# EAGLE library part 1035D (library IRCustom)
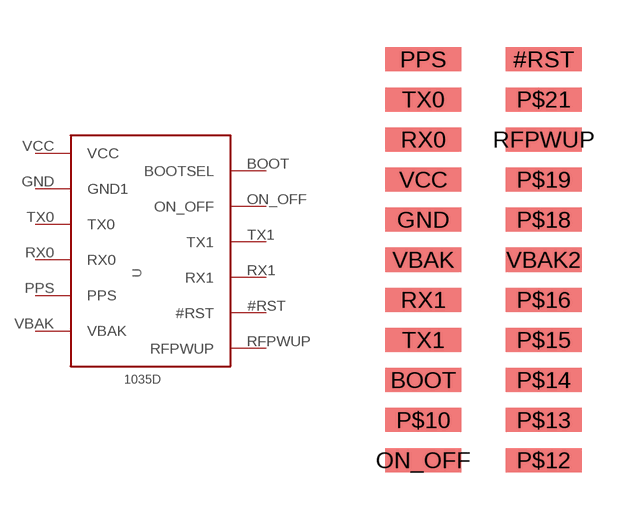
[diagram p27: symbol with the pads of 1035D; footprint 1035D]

Designator prefix -

## 1035D  [1035D]
#RST  #RST  in
BOOT  BOOTSEL  in
GND  GND1  sup
ON_OFF  ON_OFF  in
PPS  PPS  out
RFPWUP  RFPWUP  out
RX0  RX0  in
RX1  RX1  in
TX0  TX0  out
TX1  TX1  out
VBAK  VBAK  sup
VCC  VCC  sup

## Footprint 1035D (pad centres in mm)
smd 2.4 x 0.76: #RST 16.96,6.39; BOOT 13.15,-3.77; GND 13.15,1.31; ON_OFF 13.15,-6.31; P$10 13.15,-5.04; P$12 16.96,-6.31; P$13 16.96,-5.04; P$14 16.96,-3.77; P$15 16.96,-2.5; P$16 16.96,-1.23; P$18 16.96,1.31; P$19 16.96,2.58; P$21 16.96,5.12; PPS 13.15,6.39; RFPWUP 16.96,3.85; RX0 13.15,3.85; RX1 13.15,-1.23; TX0 13.15,5.12; TX1 13.15,-2.5; VBAK 13.15,0.04; VBAK2 16.96,0.04; VCC 13.15,2.58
